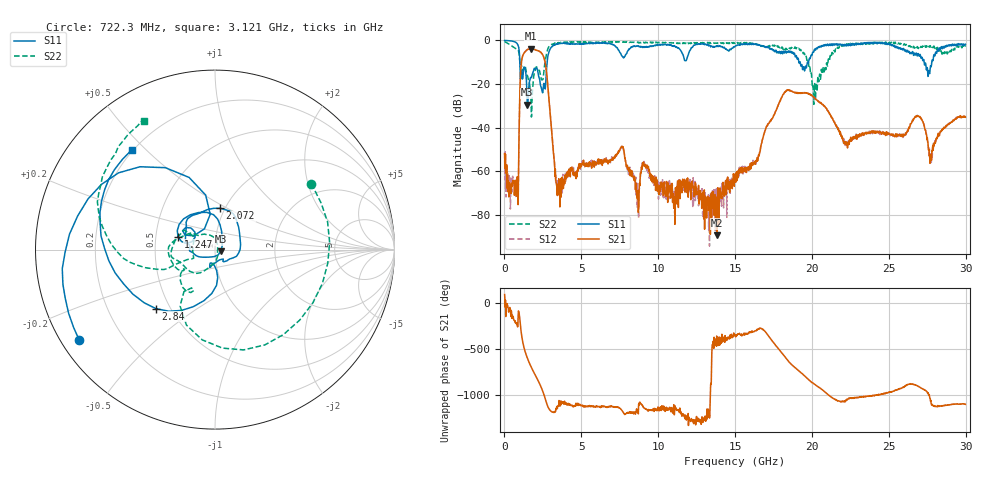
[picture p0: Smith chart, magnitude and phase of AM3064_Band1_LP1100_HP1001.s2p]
# Hz S DB R 50.0
!freq dBS11 angS11 dBS21 angS21 dBS12 angS12 dBS22 angS22
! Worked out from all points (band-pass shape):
!   1600 points, 10 MHz to 29.98 GHz, reference 50 ohm
!   highest |S21| = -3.84 dB at 1.716 GHz (marker M1); lowest = -89.3 dB at 13.82 GHz (marker M2)
!   |S21| within 3 dB of the highest: 1.198 GHz to 2.506 GHz (1.308 GHz wide, 70.6 % of centre)
!   lowest |S11| = -29.4 dB at 1.491 GHz (marker M3), VSWR 1.07, Z = 53.4 - j0.897 ohm
!   |S11| at or under -10 dB: 1.002 GHz to 2.775 GHz (1.773 GHz wide, 93.9 % of centre); 19.23 GHz to 19.71 GHz (477.2 MHz wide, 2.45 % of centre); 27.3 GHz to 27.8 GHz (495.6 MHz wide, 1.8 % of centre)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
!   |S22| runs from -35.1 to -0.5 dB; largest |S21 - S12| = 0.0082
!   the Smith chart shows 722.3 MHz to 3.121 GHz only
!   S11 on the Smith chart (normalised r, x): 722.3 MHz: 0.05, -0.30; 1.247 GHz: 0.65, +0.10; 2.072 GHz: 0.95, +0.46; 2.84 GHz: 0.42, -0.35; 3.121 GHz: 0.19, +0.45
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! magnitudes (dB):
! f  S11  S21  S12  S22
! 10 MHz  0.0  -51.9  -51.4  -0.5
! 722.3 MHz  -0.8  -65.0  -68.4  -3.7
! 1.247 GHz  -13.2  -6.1  -6.0  -12.6
! 1.491 GHz  -29.4  -4.2  -4.1  -16.1
! 1.716 GHz  -16.9  -3.8  -3.8  -26.2
! 2.072 GHz  -12.7  -4.5  -4.4  -12.2
! 2.84 GHz  -6.6  -22.5  -22.4  -3.5
! 3.121 GHz  -2.8  -45.9  -45.5  -1.7
! 3.515 GHz  -1.6  -66.6  -68.9  -1.0
! 5.015 GHz  -1.4  -57.6  -56.6  -0.7
! 7.62 GHz  -7.0  -48.8  -48.5  -0.7
! 8.651 GHz  -2.6  -72.6  -68.1  -0.9
! 10 GHz  -2.1  -67.3  -67.9  -1.0
! 13.82 GHz  -2.6  -89.3  -73.6  -1.1
! 15 GHz  -2.7  -62.1  -61.5  -1.4
! 18.25 GHz  -5.1  -23.5  -23.5  -4.3
! 19.99 GHz  -6.9  -25.2  -25.2  -17.4
! 22.18 GHz  -2.2  -47.3  -47.5  -2.2
! 25 GHz  -1.4  -42.9  -42.7  -1.1
! 26.96 GHz  -7.0  -35.0  -34.7  -3.0
! 27.73 GHz  -11.6  -54.9  -56.0  -2.9
! 29.98 GHz  -1.8  -35.2  -35.3  -2.8
